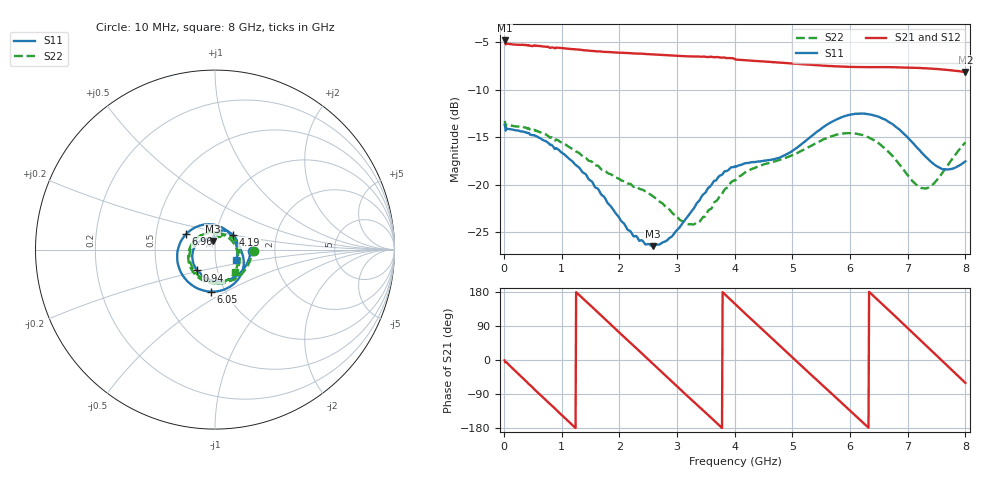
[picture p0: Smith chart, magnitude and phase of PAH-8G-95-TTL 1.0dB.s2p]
! MTS Systemtechnik GmbH
! S-Parameters
! Model: PAH-8G/95-TTL
! Attenuation Step: 1.0dB
! Rohde & Schwarz ZVB8 2Ports - Version 4.11 - 1145.1010k08 SN: 100119
! S2P File Measurements:
! S11 S21 S12 S22
# HZ  S  DB  R  50.00
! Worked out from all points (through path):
!   800 points, 10 MHz to 8 GHz, reference 50 ohm
!   highest |S21| = -4.80 dB at 10 MHz (marker M1); lowest = -8.1 dB at 8 GHz (marker M2)
!   group delay of S21, straight-line fit = 394 ps
!   lowest |S11| = -26.5 dB at 2.58 GHz (marker M3), VSWR 1.10, Z = 48.6 + j4.46 ohm
!   |S11| at or under -10 dB: start of sweep to end of sweep
!   |S22| runs from -24.2 to -13.3 dB; largest |S21 - S12| = 0.0062
!   S11 on the Smith chart (normalised r, x): 10 MHz: 1.52, -0.02; 940 MHz: 0.80, -0.19; 4.19 GHz: 1.21, +0.20; 6.05 GHz: 0.86, -0.43; 6.96 GHz: 0.71, +0.13; 8 GHz: 1.26, -0.15
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1e7  -13.66 -1.9  -4.80 -1.2  -4.72 -1.0  -13.28 -1.5
5.2e8  -14.77 -73.7  -5.32 -76.7  -5.33 -76.5  -14.21 -70.1
9.4e8  -16.28 -130.9  -5.57 -136.7  -5.56 -136.6  -15.32 -123.5
1.35e9  -18.60 177.0  -5.80 164.8  -5.80 164.8  -16.93 -171.1
1.92e9  -22.88 122.6  -6.05 83.5  -6.06 83.6  -19.19 135.2
2.28e9  -25.39 108.2  -6.17 33.0  -6.16 33.0  -20.19 109.0
2.58e9  -26.47 105.3  -6.28 -9.8  -6.27 -9.7  -21.22 88.0
2.68e9  -26.31 105.6  -6.31 -24.1  -6.31 -23.9  -21.67 82.0
3.26e9  -22.73 97.8  -6.48 -106.3  -6.49 -106.6  -24.18 67.5
3.67e9  -19.57 76.1  -6.55 -163.8  -6.53 -163.4  -21.76 66.0
4.01e9  -18.14 50.9  -6.81 146.8  -6.81 146.7  -19.54 48.1
4.19e9  -17.72 38.6  -6.88 121.4  -6.90 121.4  -18.67 36.7
4.5e9  -17.48 19.3  -7.00 77.4  -7.02 77.4  -17.85 16.5
4.85e9  -16.94 1.1  -7.16 27.8  -7.17 27.6  -17.24 -5.1
5.34e9  -14.84 -28.0  -7.38 -41.1  -7.40 -41.1  -15.86 -35.7
5.69e9  -13.35 -57.8  -7.51 -90.1  -7.52 -90.1  -14.87 -63.7
6.05e9  -12.57 -95.2  -7.59 -140.8  -7.60 -140.8  -14.58 -98.8
6.36e9  -12.61 -130.6  -7.61 175.6  -7.62 175.6  -15.13 -133.3
6.67e9  -13.38 -169.2  -7.61 131.5  -7.61 131.6  -16.56 -173.1
6.96e9  -14.77 151.4  -7.64 89.9  -7.64 89.9  -18.70 141.4
7.5e9  -18.03 61.8  -7.80 11.9  -7.80 11.8  -19.53 27.5
8e9  -17.54 -27.0  -8.12 -60.5  -8.12 -60.5  -15.53 -49.0
